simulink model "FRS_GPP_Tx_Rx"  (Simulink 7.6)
settings: Solver=FixedStepDiscrete  StartTime=0.0  StopTime=inf  RelTol=1e-3
PostLoadFcn:
  | set_param([gcs,'/usrp_helper'],'firmware','');
  | set_param([gcs,'/usrp_helper'],'bitstream','')
undefined symbols (not defined in the file or in its folder): Bit, Channels, Demo, FRS, kB, kSps, Mbit, N, RX, S, s, TX
libraries: usrp_GPP x4, dspsigops x2, simulink x2, dspsnks4 x1, dspsrcs4 x1, dspmathops x1

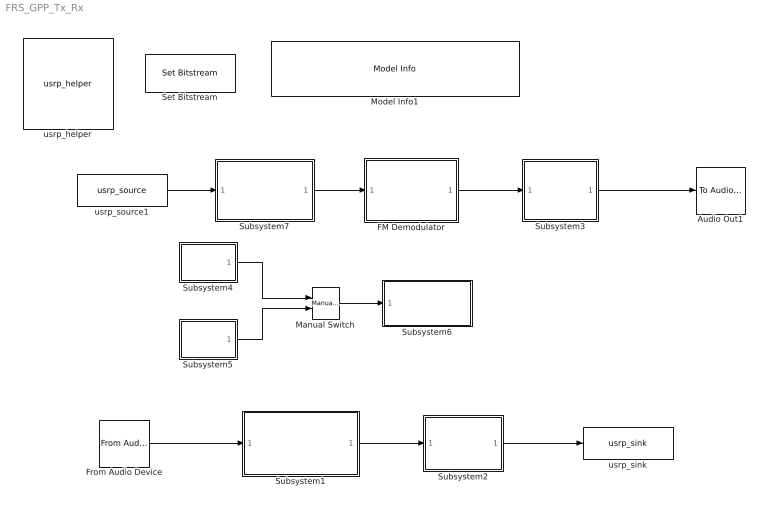
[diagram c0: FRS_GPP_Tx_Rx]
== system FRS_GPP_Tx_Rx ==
  Audio Out1 : dspsnks4/To Audio Device  DialogController=dspDDGCreate  DialogControllerArgs=DataTag0  deviceName=Default  inheritSampleRate=on  sampleRate=44100  deviceDatatype=Determine from input data type  autoBufferSize=on  bufferSize=1024  queueDuration=0.1
  FM Demodulator : Subsystem
  From Audio Device : dspsrcs4/From Audio Device  DialogController=dspDDGCreate  DialogControllerArgs=DataTag3  deviceName=Microphone (SoundMAX Integrated Digital HD Audio)  numChannels=1  sampleRate=25000  deviceDatatype=Determine from output data type  autoBufferSize=on  bufferSize=4096  queueDuration=0.1  frameSize=512  outputDatatype=single
  Manual Switch : simulink/Signal Routing/Manual Switch  SystemSampleTime=-1  sw=1  action=0  varsize=off
  Model Info1 : simulink/Model-Wide Utilities/Model Info  SystemSampleTime=-1  InitialBlockCM=None  BlockCM=None  Frame=on  DisplayStringWithTags=FRS-Demo  HorizontalTextAlignment=Center  LeftAlignmentValue=0.5  SourceBlockDiagram=FRS_GPP_Tx_Rx  TagMaxNumber=20
  Set Bitstream : usrp_GPP/Set Bitstream  SystemSampleTime=-1  bitfile=zwei.rbf
  Subsystem1 : Subsystem
  Subsystem2 : Subsystem
  Subsystem3 : Subsystem
  Subsystem4 : Subsystem
  Subsystem5 : Subsystem
  Subsystem6 : Subsystem
  Subsystem7 : Subsystem
  usrp_helper : usrp_GPP/usrp_helper  usrp_number=0  serial_number=Unknown (USRP Board #0 not found).  daughterboards_rx=Unknown (USRP Board #0 not found).  daughterboards_tx=Unknown (USRP Board #0 not found).  usb_block_size=0  usb_nblocks=0  firmware=C:\Users\nagel\Documents\sff_sdr\Simulink-USRP\simulink-usrp_2.1.0\firmware\rev4\std.ihx  bitstream=C:\Users\nagel\Documents\sff_sdr\Simulink-USRP\simulink-usrp_2.1.0\firmware\rev4\fpgaCounter.rbf  sample_time_factor=1
  usrp_sink : usrp_GPP/usrp_sink  usrp_number=0  serial_number=S/N: .  decimation=5120  sample_width=16 Bit  sampling_rate_and_bandwidth=1 Channels: 25 kSps, 97.6563 kB/s, 0.762939 Mbit/s.  vector_length=512  sideA_subdev1_tab_=0  sideA_subdev1_subdevice=Flex 2400 Tx  sideA_subdev1_datatype=SINGLE Complex  sideA_subdev1_frequency_range=Min: 2.3 GHz, Max: 2.9 GHz.  sideA_subdev1_frequency_port=off  sideA_subdev1_frequency=462.5625e6  sideA_subdev1_gain_range=Min: 0 dB, Max: 0 dB, Step Size: 1 dB.  sideA_subdev1_gain=0  sideB_subdev1_tab_=0  sideB_subdev1_subdevice=WBX NG TX  sideB_subdev1_datatype=Disabled  sideB_subdev1_frequency_range=Min: 68.75 MHz, Max: 2.2 GHz.  sideB_subdev1_frequency_port=off  sideB_subdev1_frequency=0  sideB_subdev1_gain_range=Min: 0 dB, Max: 25 dB, Step Size: 0.0223595 dB.  sideB_subdev1_gain=0
  usrp_source1 : usrp_GPP/usrp_source  usrp_number=0  serial_number=S/N: .  decimation=2560  sample_width=16 Bit  sampling_rate_and_bandwidth=1 Channels: 25 kSps, 97.6563 kB/s, 0.762939 Mbit/s.  vector_length=512  sideA_subdev1_tab_=0  sideA_subdev1_subdevice=Flex 2400 Rx  sideA_subdev1_datatype=SINGLE Complex  sideA_subdev1_frequency_range=Min: 2.3 GHz, Max: 2.9 GHz.  sideA_subdev1_frequency_port=off  sideA_subdev1_frequency=462.5625e6  sideA_subdev1_gain_range=Min: 0 dB, Max: 90 dB, Step Size: 0.05 dB.  sideA_subdev1_gain=40  sideA_subdev1_antenna=TX/RX  sideA_subdev2_tab_=0  sideA_subdev2_subdevice=Not available.  sideA_subdev2_datatype=Disabled  sideA_subdev2_frequency_range=Unknown.  sideA_subdev2_frequency_port=off  sideA_subdev2_frequency=0  sideA_subdev2_gain_range=Unknown.  sideA_subdev2_gain=0  sideB_subdev1_tab_=0  sideB_subdev1_subdevice=WBX NG RX  sideB_subdev1_datatype=Disabled  sideB_subdev1_frequency_range=Min: 68.75 MHz, Max: 2.2 GHz.  sideB_subdev1_frequency_port=off  sideB_subdev1_frequency=0  sideB_subdev1_gain_range=Min: 0 dB, Max: 50.5 dB, Step Size: 0.05 dB.  sideB_subdev1_gain=0  sideB_subdev1_antenna=Not applicable  sideB_subdev2_subdevice=Not available.  sideB_subdev2_datatype=Disabled  sideB_subdev2_frequency_range=Unknown.  sideB_subdev2_frequency_port=off  sideB_subdev2_frequency=0  sideB_subdev2_gain_range=Unknown.  sideB_subdev2_gain=0
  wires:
  usrp_source1/1 -> Subsystem7/1(In1)
  FM Demodulator/1(Out1) -> Subsystem3/1(In2)
  From Audio Device/1 -> Subsystem1/1(In1)
  Subsystem3/1(Out1) -> Audio Out1/1
  Subsystem2/1(Out1) -> usrp_sink/1
  Manual Switch/1 -> Subsystem6/1(In1)
  Subsystem4/1(Out1) -> Manual Switch/1
  Subsystem5/1(Out1) -> Manual Switch/2
  Subsystem1/1(Out1) -> Subsystem2/1(In2)
  Subsystem7/1(Out) -> FM Demodulator/1(In1)

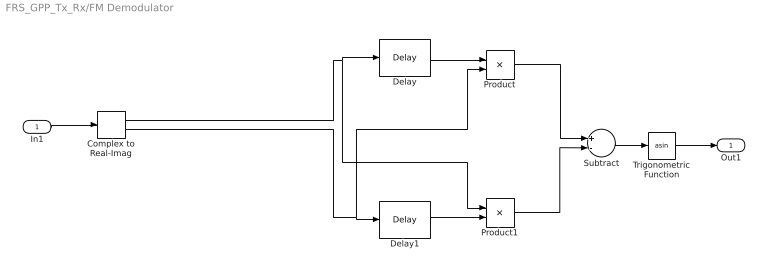
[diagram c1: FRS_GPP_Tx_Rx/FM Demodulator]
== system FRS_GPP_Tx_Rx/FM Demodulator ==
  In1 : Inport
  Complex to Real-Imag : ComplexToRealImag
  Delay : dspsigops/Delay  InputProcessing=Inherited (this choice will be removed - see release notes)  dly_unit=Samples  delay=1  ic_detail=off  dif_ic_for_ch=off  dif_ic_for_dly=off  ic=0  reset_popup=None
  Delay1 : dspsigops/Delay  InputProcessing=Inherited (this choice will be removed - see release notes)  dly_unit=Samples  delay=1  ic_detail=off  dif_ic_for_ch=off  dif_ic_for_dly=off  ic=0  reset_popup=None
  Product : Product
  Product1 : Product
  Subtract : Sum  Inputs=+-
  Trigonometric Function : Trigonometry  Operator=asin  OutputSignalType=real
  Out1 : Outport
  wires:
  Trigonometric Function/1 -> Out1/1
  In1/1 -> Complex to Real-Imag/1
  Delay/1 -> Product/1
  Subtract/1 -> Trigonometric Function/1
  Product1/1 -> Subtract/2
  Product/1 -> Subtract/1
  Delay1/1 -> Product1/2
  Complex to Real-Imag/2 -> Delay1/1, Product/2
  Complex to Real-Imag/1 -> Product1/1, Delay/1

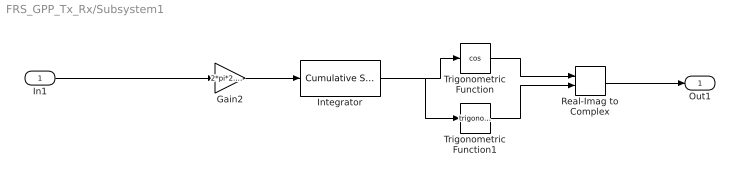
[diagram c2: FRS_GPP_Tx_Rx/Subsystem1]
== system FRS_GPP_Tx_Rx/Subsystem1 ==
  In1 : Inport
  Gain2 : Gain  Gain=2*pi*2.5e3/25e3
  Integrator : dspmathops/Cumulative Sum  DialogController=dspDDGCreate  DialogControllerArgs=DataTag5  dim=Channels (running sum)  InputProcessing=Inherited (this choice will be removed - see release notes)  reset_popup=None  outputDataTypeStr=Inherit: Same as accumulator  outputLastDataTypeStr=Inherit: Same as accumulator  outputMin=[]  outputMax=[]  roundingMode=Floor  overflowMode=off
  Real-Imag to Complex : RealImagToComplex
  Trigonometric Function : Trigonometry  Operator=cos
  Trigonometric Function1 : Trigonometry
  Out1 : Outport
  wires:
  Trigonometric Function/1 -> Real-Imag to Complex/1
  Trigonometric Function1/1 -> Real-Imag to Complex/2
  Integrator/1 -> Trigonometric Function1/1, Trigonometric Function/1
  Gain2/1 -> Integrator/1
  In1/1 -> Gain2/1
  Real-Imag to Complex/1 -> Out1/1

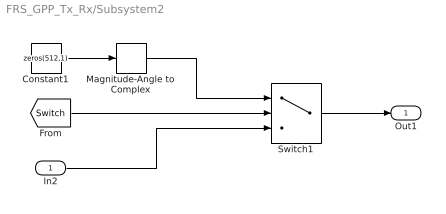
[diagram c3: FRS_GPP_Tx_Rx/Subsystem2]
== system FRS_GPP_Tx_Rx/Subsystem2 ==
  In2 : Inport
  Constant1 : Constant  Value=zeros(512,1)  VectorParams1D=off  OutDataTypeStr=single  SampleTime=1/25e3  FramePeriod=512/25e3
  Magnitude-Angle to Complex : MagnitudeAngleToComplex  Input=Magnitude
  Switch1 : Switch  Criteria=u2 > Threshold  Threshold=0.5
  Out1 : Outport
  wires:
  Constant1/1 -> Magnitude-Angle to Complex/1
  Switch1/1 -> Out1/1
  [Switch] -> Switch1/2
  Magnitude-Angle to Complex/1 -> Switch1/1
  In2/1 -> Switch1/3

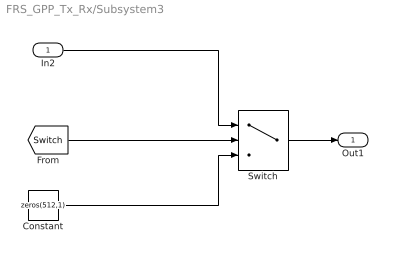
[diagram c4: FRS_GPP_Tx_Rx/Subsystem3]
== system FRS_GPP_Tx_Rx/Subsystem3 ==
  In2 : Inport
  Constant : Constant  Value=zeros(512,1)  VectorParams1D=off  SampleTime=1/25e3  FramePeriod=512/25e3
  Switch : Switch  Criteria=u2 > Threshold  Threshold=0.5
  Out1 : Outport
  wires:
  Switch/1 -> Out1/1
  In2/1 -> Switch/1
  [Switch] -> Switch/2
  Constant/1 -> Switch/3

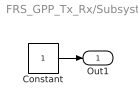
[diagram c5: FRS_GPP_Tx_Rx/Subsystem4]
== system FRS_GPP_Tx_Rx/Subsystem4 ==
  Constant : Constant  SampleTime=512/25e3
  Out1 : Outport
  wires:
  Constant/1 -> Out1/1

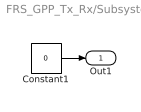
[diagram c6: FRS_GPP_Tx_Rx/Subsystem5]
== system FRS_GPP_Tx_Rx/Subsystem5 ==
  Constant1 : Constant  Value=0  SampleTime=512/25e3
  Out1 : Outport
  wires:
  Constant1/1 -> Out1/1

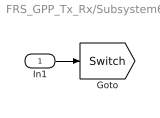
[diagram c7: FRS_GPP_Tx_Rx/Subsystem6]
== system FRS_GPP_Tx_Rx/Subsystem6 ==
  In1 : Inport
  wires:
  In1/1 -> [Switch]

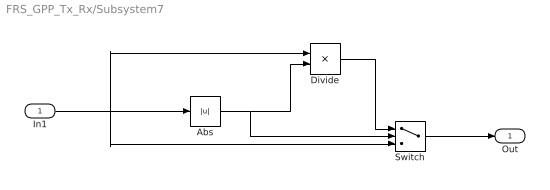
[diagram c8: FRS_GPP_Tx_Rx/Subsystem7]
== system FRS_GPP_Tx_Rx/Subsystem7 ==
  In1 : Inport
  Abs : Abs
  Divide : Product  Inputs=*/
  Switch : Switch  Criteria=u2 ~= 0
  Out : Outport
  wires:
  Abs/1 -> Divide/2, Switch/2
  Divide/1 -> Switch/1
  Switch/1 -> Out/1
  In1/1 -> Divide/1, Switch/3, Abs/1
